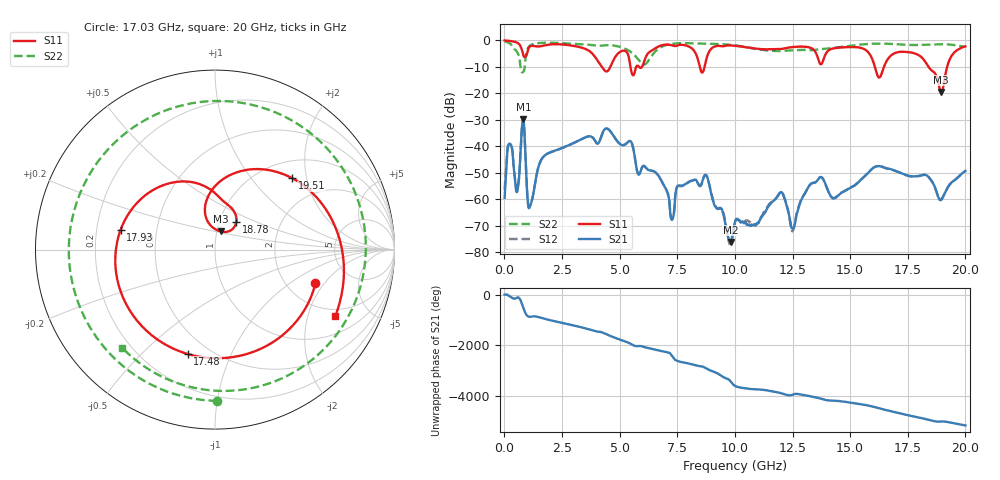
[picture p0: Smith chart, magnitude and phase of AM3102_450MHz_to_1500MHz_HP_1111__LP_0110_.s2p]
!Agilent Technologies,E8364B,MY43040894,A.07.50.67
!Agilent E8364B: A.07.50.67
!Date: Thursday, January 11, 2018 06:50:08
!Correction: S11(Full 2 Port(1,2))
!S21(Full 2 Port(1,2))
!S12(Full 2 Port(1,2))
!S22(Full 2 Port(1,2))
!S2P File: Measurements: S11, S21, S12, S22:
# Hz S  dB  R 50
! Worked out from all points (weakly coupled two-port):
!   1601 points, 10 MHz to 20 GHz, reference 50 ohm
!   highest |S21| = -29.85 dB at 822.1 MHz (marker M1); lowest = -76.0 dB at 9.818 GHz (marker M2)
!   lowest |S11| = -19.5 dB at 18.95 GHz (marker M3), VSWR 1.24, Z = 52.1 + j10.7 ohm
!   |S11| at or under -10 dB: 4.229 GHz to 4.595 GHz (365.8 MHz wide, 8.29 % of centre); 16.07 GHz to 16.47 GHz (395.8 MHz wide, 2.43 % of centre); 18.4 GHz to 19.21 GHz (809 MHz wide, 4.3 % of centre)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
!   |S22| runs from -12.1 to -0.4 dB; largest |S21 - S12| = 0.00063
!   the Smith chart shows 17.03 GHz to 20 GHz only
!   S11 on the Smith chart (normalised r, x): 17.03 GHz: 2.84, -1.64; 17.48 GHz: 0.38, -0.70; 17.93 GHz: 0.30, +0.09; 18.78 GHz: 1.20, +0.38; 19.51 GHz: 1.36, +1.65; 20 GHz: 1.68, -3.01
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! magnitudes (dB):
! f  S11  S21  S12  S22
! 10 MHz  -0.1  -59.4  -56.3  -0.4
! 234.9 MHz  -0.3  -39.0  -39.0  -1.1
! 559.7 MHz  -0.9  -57.1  -56.7  -4.6
! 822.1 MHz  -5.6  -29.9  -29.9  -11.9
! 1.109 GHz  -2.3  -62.5  -62.5  -2.0
! 3.346 GHz  -2.8  -37.3  -37.2  -1.5
! 6.682 GHz  -2.4  -51.0  -51.1  -3.2
! 7.281 GHz  -2.0  -67.6  -67.3  -1.3
! 8.756 GHz  -7.3  -50.9  -50.9  -1.3
! 9.818 GHz  -1.9  -76.0  -77.6  -1.7
! 10.01 GHz  -2.1  -68.5  -68.6  -1.9
! 11.99 GHz  -3.3  -57.2  -57.2  -4.0
! 12.52 GHz  -2.6  -71.0  -71.9  -3.8
! 13.34 GHz  -3.1  -53.9  -53.9  -3.7
! 16.68 GHz  -6.6  -48.5  -48.5  -1.3
! 17.03 GHz  -4.6  -49.5  -49.4  -1.5
! 17.48 GHz  -4.4  -51.0  -51.0  -1.7
! 17.93 GHz  -5.4  -51.2  -51.2  -1.8
! 18.78 GHz  -14.3  -58.1  -57.8  -1.5
! 18.95 GHz  -19.5  -60.2  -59.9  -1.5
! 19.51 GHz  -4.6  -52.8  -52.9  -1.8
! 20 GHz  -2.3  -49.3  -49.3  -2.5
